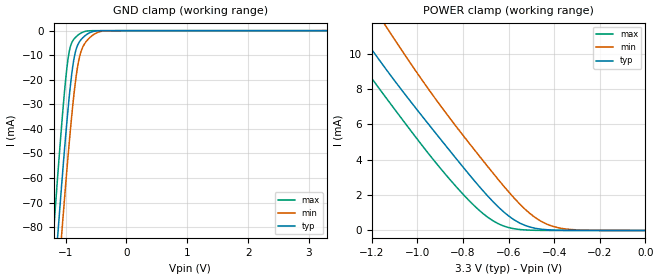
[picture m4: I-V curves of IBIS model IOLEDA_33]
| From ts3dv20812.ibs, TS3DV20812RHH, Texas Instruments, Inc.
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[Model]   IOLEDA_33
Model_type  Terminator
| variable   typ   min   max
C_comp   8.18pF   6.94pF   9.38pF
| C_tri-state   8.18pF   6.94pF   9.38pF
[Temperature Range]   40   100   -40
| Ambient temperature   25   85   -40
[Voltage range]   3.3   3   3.6
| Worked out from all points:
|   GND clamp passes 1 mA (typ) near -0.62 V on its own axis
|   POWER clamp passes 1 mA (typ) near -0.62 V on its own axis
[GND Clamp]
| TS3DV20812_IOLEDA_33
|   Voltage   I(typ)   I(min)   I(max)
-3.3V     -860.8mA   -867.9mA   -859mA
-1.205V   -108.2mA   -128.4mA   -84.08mA
-1.135V   -84.87mA   -105.2mA   -60.39mA
-1.12V    -79.97mA   -100.3mA   -55.45mA
-1.065V   -62.39mA   -82.7mA    -38.02mA
-950mV    -29.07mA   -47.99mA   -9.716mA
-855mV    -10.35mA   -23.97mA   -3.174mA
-800mV    -5.712mA   -14.12mA   -1.864mA
-735mV    -3.311mA   -7.63mA    -813.6uA
-555mV    -388.1uA   -1.84mA    -10.57uA
-335mV    -2.028uA   -62.42uA   -2.508nA
3.3V      5.2nA      32.32uA    3.428nA
[POWER Clamp]
| TS3DV20812_IOLEDA_33
|   Voltage   I(typ)   I(min)   I(max)
-3.3V     45.11mA    47.13mA    47.54mA
-1.355V   13.11mA    16.04mA    11.48mA
-1.255V   11.23mA    13.92mA    9.587mA
-1.15V    9.336mA    11.79mA    7.72mA
-1.12V    8.813mA    11.19mA    7.2mA
-930mV    5.667mA    7.608mA    4mA
-775mV    3.195mA    4.969mA    1.71mA
-670mV    1.649mA    3.268mA    559.5uA
-575mV    595.5uA    1.821mA    96.04uA
-480mV    116.9uA    700.9uA    8.897uA
-385mV    15.36uA    162.8uA    589.9nA
0V        0A         0A         0A
